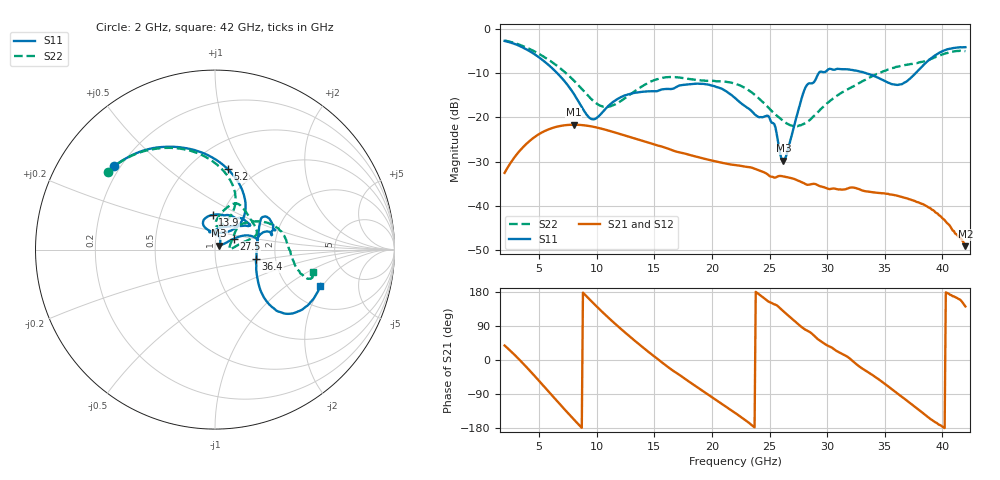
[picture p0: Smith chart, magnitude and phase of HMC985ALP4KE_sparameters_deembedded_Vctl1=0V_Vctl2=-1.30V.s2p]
!s2p File: Measurements: S11, S21, S12, S22
# GHz S dB R 50.0
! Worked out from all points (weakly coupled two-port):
!   401 points, 2 GHz to 42 GHz, reference 50 ohm
!   highest |S21| = -21.68 dB at 8 GHz (marker M1); lowest = -49.1 dB at 42 GHz (marker M2)
!   lowest |S11| = -29.8 dB at 26.2 GHz (marker M3), VSWR 1.07, Z = 52.4 + j2.29 ohm
!   |S11| at or under -10 dB: 6.561 GHz to 29.27 GHz (22.71 GHz wide, 127 % of centre); 33.35 GHz to 37.69 GHz (4.343 GHz wide, 12.2 % of centre)
!   |S22| runs from -22.0 to -2.6 dB; largest |S21 - S12| = 0.00017
!   S11 on the Smith chart (normalised r, x): 2 GHz: 0.18, +0.35; 5.2 GHz: 0.75, +0.84; 13.9 GHz: 0.90, +0.36; 27.5 GHz: 1.22, +0.15; 36.4 GHz: 1.58, -0.18; 42 GHz: 2.90, -1.91
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2  -2.74 140.6  -32.58 38.2  -32.58 38.2  -2.63 144.0
3.5  -4.12 112.9  -27.04 -5.9  -27.04 -5.9  -3.80 119.1
5.2  -6.87 80.9  -23.49 -62.2  -23.49 -62.2  -5.99 93.1
8  -14.67 46.0  -21.68 -156.5  -21.69 -156.5  -11.67 65.2
8.7  -17.70 51.9  -21.76 -179.0  -21.77 -179.0  -13.60 65.0
9.7  -20.47 85.0  -22.14 150.0  -22.14 149.9  -16.31 72.0
10.9  -17.72 113.4  -22.92 114.7  -22.92 114.7  -17.65 85.7
13.9  -14.26 93.9  -25.26 35.8  -25.25 35.8  -13.05 77.6
15.4  -13.94 73.0  -26.45 -0.0  -26.46 -0.0  -11.26 68.5
19.4  -12.52 34.5  -29.41 -85.9  -29.42 -85.9  -11.73 37.0
22  -15.62 52.3  -30.80 -139.4  -30.81 -139.4  -12.40 19.1
25  -20.17 98.0  -33.28 152.7  -33.29 152.8  -18.09 10.3
26.2  -29.79 42.3  -33.38 128.5  -33.37 128.5  -20.88 3.2
27.5  -18.39 29.9  -34.34 93.9  -34.31 93.8  -21.92 6.5
28.1  -13.35 20.8  -35.07 80.1  -35.07 80.0  -21.34 14.9
28.7  -12.31 12.9  -35.08 68.9  -35.09 68.7  -20.10 24.0
31  -9.08 23.4  -36.34 21.0  -36.31 20.9  -14.85 44.3
33.3  -9.96 34.4  -36.72 -27.1  -36.72 -27.1  -11.55 36.3
35.4  -12.27 12.3  -37.42 -72.1  -37.39 -71.8  -9.13 23.0
36.4  -12.57 -12.9  -37.98 -95.1  -37.97 -95.2  -8.35 15.5
39.5  -5.81 -43.3  -41.66 -165.8  -41.62 -166.1  -6.28 -14.4
42  -4.15 -19.0  -49.14 141.3  -48.95 142.1  -5.05 -12.8
